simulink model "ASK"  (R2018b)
settings: Solver=VariableStepAuto  StartTime=0.0  StopTime=20  FixedStep=1e-5  RelTol=1e-3
libraries: commdigbbndam3 x2, commchan3 x1, commrandsrc3 x1, dspsrcs4 x1

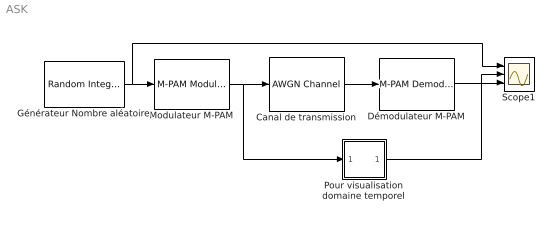
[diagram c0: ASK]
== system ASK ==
  Canal de transmission : commchan3/AWGN Channel  InputProcessing=Columns as channels (frame based)  seed=67  noiseMode="Signal to noise ratio  (SNR)"  EbNodB=40  EsNodB=10  SNRdB=30  bitsPerSym=8  Ps=1  Tsym=1/100000  variance=1
  Démodulateur M-PAM : commdigbbndam3/M-PAM Demodulator Baseband  M=8  OutType=Integer  Dec=Binary  PowType=Min. distance between symbols  MinDist=2  AvgPow=1  PeakPow=1  outDtype1=Inherit via internal rule  outDtype2=Inherit via internal rule  denormFactorWordLen=16  denormFactorDataTypeStr=Inherit: Same word length as input  denormFactorLastDataTypeStr=Inherit: Same word length as input  prodOutWordLen=16  prodOutRoundingMode=Floor  prodOutOverflowMode=Wrap  prodOutOvFlMode=off  prodOutOvFlModeLastStrValue=off  sumWordLen=16
  Générateur Nombre aléatoire : commrandsrc3/Random Integer Generator  SetSize=8  SeedSource=Auto  Seed=0  SampleTime=1  SamplesPerFrame=1  OutputDataType=double  SimulateUsing=Interpreted execution
  Modulateur M-PAM : commdigbbndam3/M-PAM Modulator Baseband  M=8  InType=Integer  Enc=Binary  PowType=Min. distance between symbols  MinDist=2  AvgPow=1  PeakPow=1  outDtype=double  outWordLen=16  outUDDataType=sfix(16)  outFracLenMode=Best precision  outFracLen=15  outDataTypeStr=double  outLastDataTypeStr=double
  Pour visualisation domaine temporel : Subsystem
  Scope1 : Scope  NumInputPorts=3
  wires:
  Modulateur M-PAM/1 -> Pour visualisation domaine temporel/1(In1), Canal de transmission/1
  Canal de transmission/1 -> Démodulateur M-PAM/1
  Générateur Nombre aléatoire/1 -> Modulateur M-PAM/1, Scope1/1
  Démodulateur M-PAM/1 -> Scope1/3
  Pour visualisation domaine temporel/1(Out1) -> Scope1/2

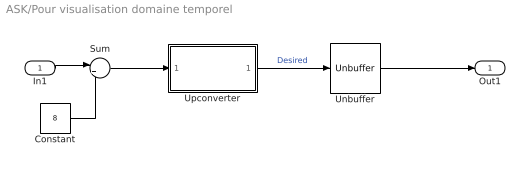
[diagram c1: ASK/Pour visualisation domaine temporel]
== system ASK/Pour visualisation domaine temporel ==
  In1 : Inport
  Constant : Constant  Value=8
  Sum : Sum  Inputs=|++
  Unbuffer : Unbuffer
  Upconverter : Subsystem
  Out1 : Outport
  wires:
  Constant/1 -> Sum/2
  Sum/1 -> Upconverter/1(In)
  Unbuffer/1 -> Out1/1
  Upconverter/1(Out) -> Unbuffer/1  "Desired"
  In1/1 -> Sum/1

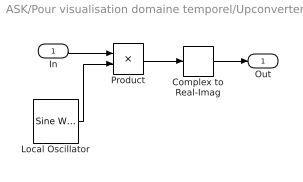
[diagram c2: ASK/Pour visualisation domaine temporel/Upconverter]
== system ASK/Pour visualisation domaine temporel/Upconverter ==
  In : Inport
  Complex to Real-Imag : ComplexToRealImag  Output=Real
  Local Oscillator : dspsrcs4/Sine Wave  Amplitude=1  Frequency=20  Phase=0  SampleMode=Discrete  OutComplex=Complex  CompMethod=Trigonometric fcn  TableSize=Speed  SampleTime=1/100000  SamplesPerFrame=100000  ResetState=Restart at time zero  OutputFrames=off  dataType=double  wordLen=16  udDataType=sfix(16)  fracBitsMode=Best precision  numFracBits=15  OutDataTypeStr=double  LastOutDataTypeStr=double
  Product : Product
  Out : Outport
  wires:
  Complex to Real-Imag/1 -> Out/1
  Product/1 -> Complex to Real-Imag/1
  Local Oscillator/1 -> Product/2
  In/1 -> Product/1
